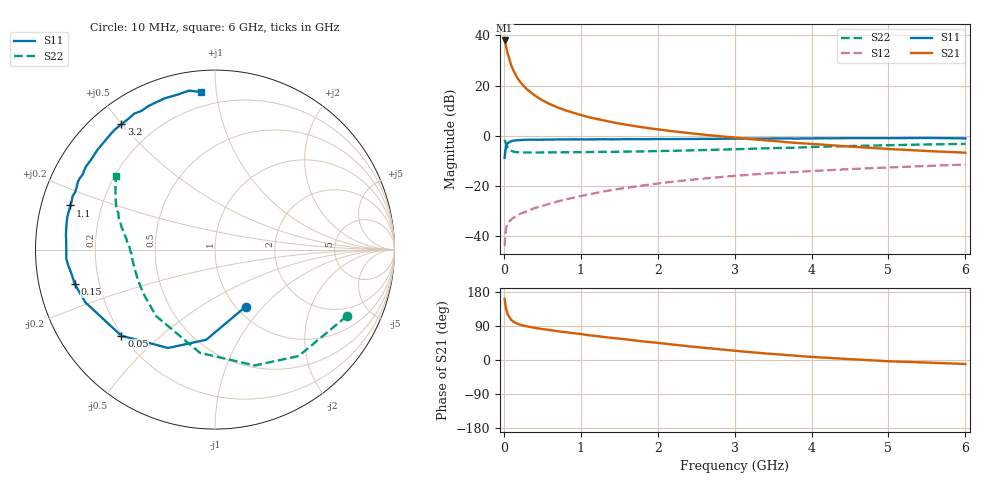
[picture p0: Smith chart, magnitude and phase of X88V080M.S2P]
! SIEMENS Small Signal Semiconductors
! BFP136W
! Si NPN RF Bipolar Junction Transistor in SOT343
! VCE = 8 V  IC = 80 mA
! Common Emitter S-Parameters:  September  1994
# GHz  S  MA  R  50
!  f  S11  S21  S12  S22
! GHz  MAG  ANG  MAG  ANG  MAG  ANG  MAG  ANG
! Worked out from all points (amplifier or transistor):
!   40 points, 10 MHz to 6 GHz, reference 50 ohm
!   highest |S21| = 38.0 dB at 10 MHz (marker M1)
!   |S21| within 3 dB of that: start of sweep to 33.51 MHz
!   unconditionally stable (mu >= 1): 707.4 MHz to 2.971 GHz
!   at 200 MHz: K = 0.61, MSG = 26.7 dB, |S12| = -31.4 dB
!   at 1.5 GHz: K = 1.10, MAG = 11.1 dB, |S12| = -21.2 dB
!   at 6 GHz: K = 0.96, MSG = 2.4 dB, |S12| = -11.6 dB
!   S11 on the Smith chart (normalised r, x): 10 MHz: 1.10, -0.81; 50 MHz: 0.20, -0.38; 150 MHz: 0.11, -0.12; 1.1 GHz: 0.09, +0.15; 3.2 GHz: 0.09, +0.50; 6 GHz: 0.12, +0.91
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0.01  0.3607 -61.8  79.55 161.5  0.0062 68.8  0.8224 -26.8
0.02  0.5044 -95.5  69.33 146.0  0.011 58.7  0.7544 -51.8
0.03  0.6073 -115.5  59.55 134.5  0.0142 51.6  0.6824 -71.1
0.05  0.7089 -137.4  43.32 120.1  0.018 40.0  0.5813 -98.3
0.1  0.7796 -157.8  24.33 104.9  0.0216 36.0  0.4946 -131.6
0.15  0.8044 -166.1  16.61 98.1  0.0242 36.9  0.4698 -146.1
0.2  0.8115 -170.6  12.52 94.0  0.0269 38.3  0.4629 -154.1
0.25  0.8225 -173.9  10.1 91.0  0.029 39.7  0.4613 -159.2
0.3  0.8301 -176.4  8.457 88.8  0.0308 41.4  0.4593 -162.6
0.4  0.8287 179.4  6.374 84.9  0.0357 44.5  0.4607 -167.3
0.5  0.8307 176.5  5.086 81.6  0.0395 47.1  0.4618 -170.5
0.6  0.8351 174.1  4.25 79.0  0.0438 49.1  0.4629 -172.6
0.7  0.8377 171.5  3.661 75.9  0.0485 51.6  0.4641 -174.1
0.9  0.8427 167.6  2.866 70.9  0.0574 53.3  0.4662 -176.8
1.1  0.842 163.0  2.345 65.4  0.0669 54.8  0.4703 -178.6
1.5  0.8444 156.1  1.745 56.3  0.0866 55.3  0.4768 178.3
1.8  0.8475 150.3  1.469 49.3  0.101 54.3  0.4842 176.0
2.2  0.8532 143.8  1.221 40.7  0.1202 52.2  0.4973 173.1
3.2  0.8718 126.7  0.853 20.8  0.1654 44.4  0.5448 164.7
4.5  0.8885 108.6  0.605 2.3  0.2146 33.8  0.6191 153.3
5.5  0.8978 99.3  0.493 -6.8  0.2476 25.7  0.6666 146.4
6  0.8812 95.0  0.456 -10.5  0.2644 21.5  0.6845 143.4
